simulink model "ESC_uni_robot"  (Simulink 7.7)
settings: Solver=ode3  StartTime=starttime  StopTime=stoptime  FixedStep=stepsize  RelTol=1e-3
PreLoadFcn:
  | load('ESC_GUI_params_uni')
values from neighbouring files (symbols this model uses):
  Kd = 60    [sim_run_multi.m]    (also in sim_run_uni.m)
  Kp = 3000    [sim_run_multi.m]    (also in sim_run_uni.m)
  noise_max = value    [ESC_GUI_multi.m]    (also in ESC_GUI_uni.m; sim_run_multi.m = 0.01; sim_run_uni.m = 0.2)
  obj_mean = -0.4    [sim_run_uni.m]
  obj_var = 0.27    [sim_run_uni.m]
  switch_noise = 1    [ESC_GUI_multi.m]    (also in ESC_GUI_uni.m; sim_run_multi.m; sim_run_uni.m)
  switch_optimizer = method_no+1    [ESC_GUI_multi.m]    (also in ESC_GUI_uni.m = method_no; sim_run_multi.m = 4; sim_run_uni.m = 1)
  x0 = [0;0]    [sim_run_multi.m]    (also in sim_run_uni.m = 0)
undefined symbols (not defined in the file or in its folder): approx, nn, perturb, sm_periodic
libraries: roblocks x8, simulink x1, commnoisgen2 x1

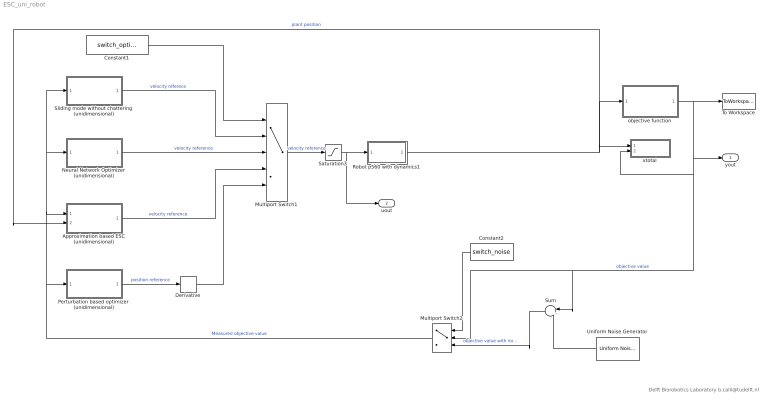
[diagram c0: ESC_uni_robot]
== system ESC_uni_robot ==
  note: Delft Biorobotics Laboratory b.calli@tudelft.nl
  Approximation based ESC (unidimensional) : Subsystem  mask{K_grad=approx.K_grad, sampling=approx.sampling, data_size=approx.data_size, poly_degree=approx.poly_degree, vel_init=approx.vel_init, lpf_constant=approx.filter_constant}
      mask prompts: data_size "Data size"; poly_degree "Poly degree"; vel_init "Initial velocity"; lpf_constant "Filter Constant"
  Constant1 : Constant  Value=switch_optimizer
  Constant2 : Constant  Value=switch_noise
  Derivative : Derivative
  Multiport Switch1 : MultiPortSwitch  Inputs=4  zeroidx=off
  Multiport Switch2 : MultiPortSwitch  Inputs=2  zeroidx=off
  Neural Network Optimizer (unidimensional) : Subsystem  mask{M=nn.M, A=nn.A, B=nn.B, ddelta=nn.ddelta, delta=nn.delta, mpd_init=nn.mpd_init}
      mask prompts: mpd_init "Minimum peak detector initial value"
  Perturbation based optimizer (unidimensional) : Subsystem  mask{high_pass_pole=perturb.high_pass_pole, sine_amp=perturb.sine_amp, sine_freq=perturb.sine_freq, low_pass_pole=perturb.low_pass_pole, corr_gain=perturb.corr_gain, comp_zero=perturb.comp_zero, comp_pole=perturb.comp_pole}
      mask prompts: high_pass_pole "High Pass Filter Pole"; sine_amp "Perturbation Signal Amplitude"; sine_freq "Perturbation Signal Frequency"; low_pass_pole "Low Pass Filter Pole"; corr_gain "Correction Gain"; comp_zero "Compensator Zero"; comp_pole "Compensator Pole"
  Robot p560 with dynamics1 : Subsystem
  Saturation3 : Saturate  UpperLimit=1  LowerLimit=-1
  Sliding mode without chattering (unidimensional) : Subsystem  mask{alpha=sm_periodic.alpha, rho=sm_periodic.rho, k=sm_periodic.k, g_init=sm_periodic.g_init}
      mask prompts: g_init "initial g"
  Sum : Sum  Inputs=|++
  To Workspace : ToWorkspace  VariableName=y  SampleTime=-1  SaveFormat=Structure With Time
  Uniform Noise Generator : commnoisgen2/Uniform Noise Generator  SystemSampleTime=-1  low=-noise_max  up=noise_max  seed=31  Ts=0.001  frameBased=off  sampPerFrame=1  orient=off  outDataType=double
  objective function : Stateflow chart  TreatAsAtomicUnit=on
  xtotal : Subsystem
  yout : Outport
  uout : Outport  Port=2
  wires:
  Robot p560 with dynamics1/1(x) -> objective function/1(x), Approximation based ESC (unidimensional)/2(x), xtotal/1(x)  "plant position"
  Multiport Switch1/1 -> Saturation3/1  "velocity reference"
  Neural Network Optimizer (unidimensional)/1(xdot_ref) -> Multiport Switch1/3  "velocity reference"
  Sliding mode without chattering (unidimensional)/1(xdot_ref) -> Multiport Switch1/2  "velocity referece"
  Constant1/1 -> Multiport Switch1/1
  Approximation based ESC (unidimensional)/1(xdot_ref) -> Multiport Switch1/4  "velocity reference"
  objective function/1(y) -> To Workspace/1, Multiport Switch2/2, Sum/1, xtotal/2(y), yout/1  "objective value"
  Uniform Noise Generator/1 -> Sum/2
  Sum/1 -> Multiport Switch2/3  "objective value with noise"
  Constant2/1 -> Multiport Switch2/1
  Perturbation based optimizer (unidimensional)/1(xref) -> Derivative/1  "position reference"
  Derivative/1 -> Multiport Switch1/5
  Multiport Switch2/1 -> Sliding mode without chattering (unidimensional)/1(y), Neural Network Optimizer (unidimensional)/1(y), Approximation based ESC (unidimensional)/1(y), Perturbation based optimizer (unidimensional)/1(y)  "Measured objective value"
  Saturation3/1 -> Robot p560 with dynamics1/1(xref), uout/1

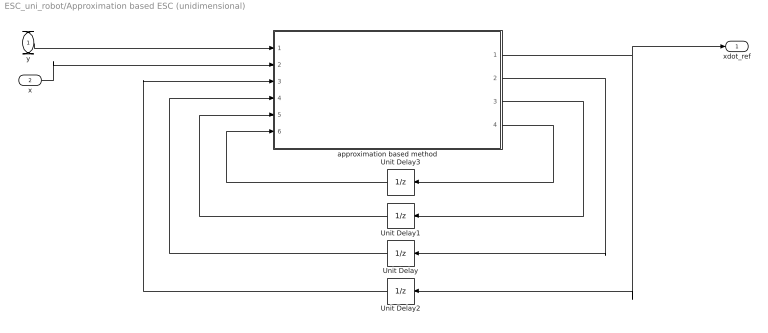
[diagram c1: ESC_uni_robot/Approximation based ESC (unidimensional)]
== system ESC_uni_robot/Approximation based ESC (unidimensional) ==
  y : Inport
  x : Inport  Port=2
  Unit Delay : UnitDelay  X0=zeros(1,data_size)  SampleTime=-1
  Unit Delay1 : UnitDelay  X0=zeros(1,data_size)  SampleTime=-1
  Unit Delay2 : UnitDelay  SampleTime=-1
  Unit Delay3 : UnitDelay  SampleTime=-1
  approximation based method : Stateflow chart  TreatAsAtomicUnit=on
  xdot_ref : Outport
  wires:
  approximation based method/2(x_data_arr_out) -> Unit Delay/1
  Unit Delay/1 -> approximation based method/4(x_data_arr)
  approximation based method/3(y_data_arr_out) -> Unit Delay1/1
  Unit Delay1/1 -> approximation based method/5(y_data_arr)
  y/1 -> approximation based method/1(y_data_in)
  x/1 -> approximation based method/2(x_data_in)
  approximation based method/1(xdot_ref) -> Unit Delay2/1, xdot_ref/1
  approximation based method/4(sample_out) -> Unit Delay3/1
  Unit Delay2/1 -> approximation based method/3(xdot_ref_in)
  Unit Delay3/1 -> approximation based method/6(sample)

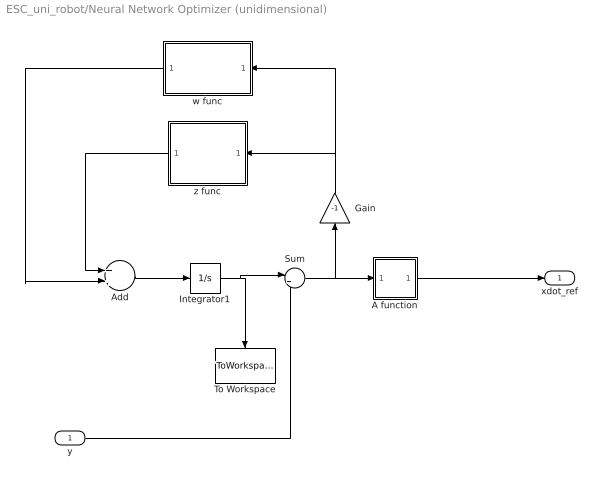
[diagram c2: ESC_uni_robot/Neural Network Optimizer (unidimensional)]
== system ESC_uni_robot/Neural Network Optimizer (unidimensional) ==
  y : Inport
  A function : Subsystem
  Add : Sum
  Gain : Gain  Gain=-1
  Integrator1 : Integrator  InitialCondition=mpd_init
  Sum : Sum  Inputs=|+-
  To Workspace : ToWorkspace  VariableName=yd_out  SampleTime=-1  SaveFormat=Structure With Time
  w func : Subsystem
  z func : Subsystem
  xdot_ref : Outport
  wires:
  Sum/1 -> Gain/1, A function/1(e)
  Gain/1 -> w func/1(e_minus), z func/1(e_minus)
  w func/1(w) -> Add/2
  z func/1(z) -> Add/1
  Add/1 -> Integrator1/1
  Integrator1/1 -> Sum/1, To Workspace/1
  A function/1(xdot) -> xdot_ref/1
  y/1 -> Sum/2

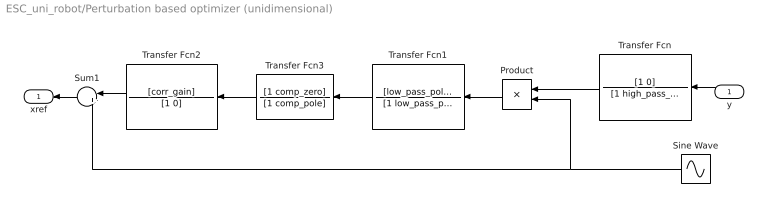
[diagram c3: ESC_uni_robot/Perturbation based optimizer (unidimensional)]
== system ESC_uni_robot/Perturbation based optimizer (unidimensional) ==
  y : Inport
  Product : Product
  Sine Wave : Sin  Amplitude=sine_amp  Frequency=sine_freq  SampleTime=0
  Sum1 : Sum  Inputs=|++
  Transfer Fcn : TransferFcn  Numerator=[1 0]  Denominator=[1 high_pass_pole]
  Transfer Fcn1 : TransferFcn  Numerator=[low_pass_pole]  Denominator=[1 low_pass_pole]
  Transfer Fcn2 : TransferFcn  Numerator=[corr_gain]  Denominator=[1 0]
  Transfer Fcn3 : TransferFcn  Numerator=[1 comp_zero]  Denominator=[1 comp_pole]
  xref : Outport
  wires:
  Transfer Fcn/1 -> Product/1
  Sine Wave/1 -> Product/2, Sum1/2
  Product/1 -> Transfer Fcn1/1
  Transfer Fcn1/1 -> Transfer Fcn3/1
  Transfer Fcn2/1 -> Sum1/1
  y/1 -> Transfer Fcn/1
  Sum1/1 -> xref/1
  Transfer Fcn3/1 -> Transfer Fcn2/1

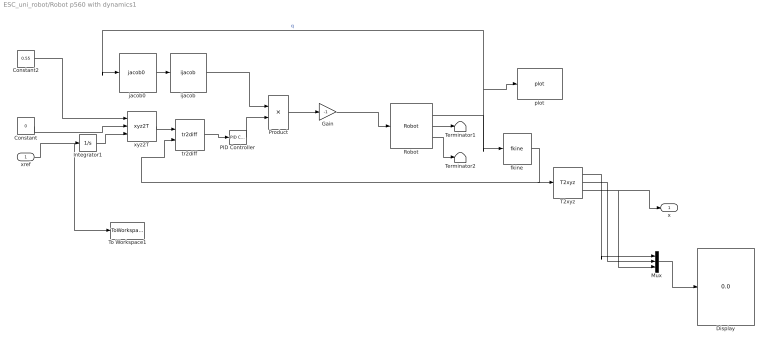
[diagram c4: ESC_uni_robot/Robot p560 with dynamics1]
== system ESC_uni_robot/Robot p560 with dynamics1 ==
  xref : Inport
  Constant : Constant  Value=0
  Constant2 : Constant  Value=0.55
  Display : Display
  Gain : Gain  Gain=-1
  Integrator1 : Integrator  InitialCondition=x0
  Mux : Mux  Inputs=3
  PID Controller : simulink/Continuous/PID Controller  SystemSampleTime=-1  Controller=PID  TimeDomain=Continuous-time  SampleTime=1  IntegratorMethod=Forward Euler  FilterMethod=Forward Euler  Form=Parallel  P=[Kp Kp Kp Kp Kp Kp]  I=[0 0 0 0 0 0]  D=[Kd Kd Kd Kd Kd Kd]  N=100  InitialConditionSource=internal  InitialConditionForIntegrator=0  InitialConditionForFilter=0  ExternalReset=none  LimitOutput=off  UpperSaturationLimit=inf  LowerSaturationLimit=-inf  LinearizeAsGain=off  AntiWindupMode=none  Kb=1  TrackingMode=off  Kt=1  PParamMin=[]  PParamMax=[]  IParamMin=[]  IParamMax=[]  DParamMin=[]  DParamMax=[]  NParamMin=[]  NParamMax=[]  KbParamMin=[]  KbParamMax=[]  KtParamMin=[]  KtParamMax=[]  POutMin=[]  POutMax=[]  IOutMin=[]  IOutMax=[]  DOutMin=[]  DOutMax=[]  NOutMin=[]  NOutMax=[]  KbOutMin=[]  KbOutMax=[]  KtOutMin=[]  KtOutMax=[]  IntegratorOutMin=[]  IntegratorOutMax=[]  FilterOutMin=[]  FilterOutMax=[]  SumOutMin=[]  SumOutMax=[]  SumI1OutMin=[]  SumI1OutMax=[]  SumI2OutMin=[]  SumI2OutMax=[]  SumI3OutMin=[]  SumI3OutMax=[]  SumDOutMin=[]  SumDOutMax=[]  SaturationOutMin=[]  SaturationOutMax=[]  IntegratorContinuousStateAttributes=''  IntegratorStateMustResolveToSignalObject=off  IntegratorRTWStateStorageClass=Auto  FilterContinuousStateAttributes=''  FilterStateMustResolveToSignalObject=off  FilterRTWStateStorageClass=Auto
  Product : Product  Multiplication=Matrix(*)
  Robot : roblocks/Robot  SystemSampleTime=-1  robot=p560  q0="[0.2763    0.9125    2.9359         0    2.4348   -0.2763]"
  T2xyz : roblocks/T2xyz  SystemSampleTime=-1
  Terminator1 : Terminator
  Terminator2 : Terminator
  To Workspace1 : ToWorkspace  VariableName=u_out  SampleTime=-1  SaveFormat=Structure With Time
  fkine : roblocks/fkine  SystemSampleTime=-1  robot=p560
  ijacob : roblocks/ijacob  SystemSampleTime=-1
  jacob0 : roblocks/jacob0   SystemSampleTime=-1  robot=p560
  plot : roblocks/plot  SystemSampleTime=-1  robot=p560
  tr2diff : roblocks/tr2diff  SystemSampleTime=-1  robot=robot
  xyz2T : roblocks/xyz2T  SystemSampleTime=-1
  x : Outport
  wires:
  Robot/1 -> fkine/1, jacob0/1, plot/1  "q"
  tr2diff/1 -> PID Controller/1
  xyz2T/1 -> tr2diff/1
  fkine/1 -> T2xyz/1, tr2diff/2
  jacob0/1 -> ijacob/1
  ijacob/1 -> Product/1
  Product/1 -> Gain/1
  Gain/1 -> Robot/1
  PID Controller/1 -> Product/2
  Robot/2 -> Terminator1/1
  Robot/3 -> Terminator2/1
  xref/1 -> Integrator1/1, To Workspace1/1
  T2xyz/1 -> Mux/1
  T2xyz/2 -> Mux/2
  T2xyz/3 -> Mux/3, x/1
  Mux/1 -> Display/1
  Constant/1 -> xyz2T/2
  Constant2/1 -> xyz2T/1
  Integrator1/1 -> xyz2T/3

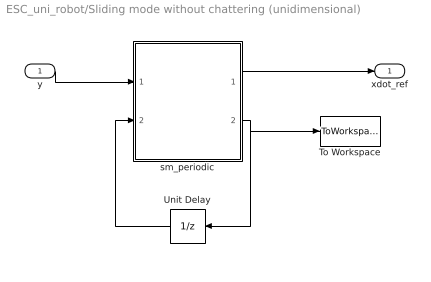
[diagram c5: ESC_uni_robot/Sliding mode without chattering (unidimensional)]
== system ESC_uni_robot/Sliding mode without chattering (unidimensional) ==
  y : Inport
  To Workspace : ToWorkspace  VariableName=g_sm_out  SampleTime=-1  SaveFormat=Structure With Time
  Unit Delay : UnitDelay  X0=g_init  SampleTime=-1
  sm_periodic : Stateflow chart  TreatAsAtomicUnit=on
  xdot_ref : Outport
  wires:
  y/1 -> sm_periodic/1(y)
  sm_periodic/1(u) -> xdot_ref/1
  sm_periodic/2(g_out) -> Unit Delay/1, To Workspace/1
  Unit Delay/1 -> sm_periodic/2(g_in)

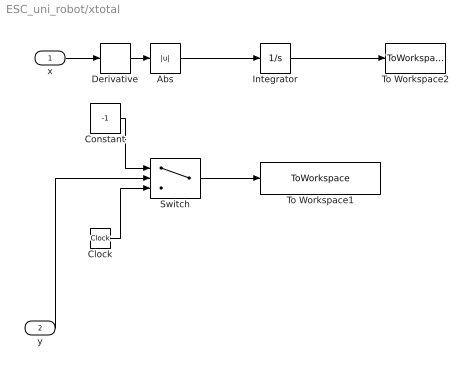
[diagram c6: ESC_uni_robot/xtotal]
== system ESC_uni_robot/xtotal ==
  x : Inport
  y : Inport  Port=2
  Abs : Abs
  Clock : Clock
  Constant : Constant  Value=-1
  Derivative : Derivative
  Integrator : Integrator
  Switch : Switch  Threshold=1.05
  To Workspace1 : ToWorkspace  VariableName=peak_time_detector  SampleTime=-1  SaveFormat=Array
  To Workspace2 : ToWorkspace  VariableName=x_total  SampleTime=-1  SaveFormat=Array
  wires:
  y/1 -> Switch/2
  Clock/1 -> Switch/3
  Switch/1 -> To Workspace1/1
  Constant/1 -> Switch/1
  x/1 -> Derivative/1
  Integrator/1 -> To Workspace2/1
  Abs/1 -> Integrator/1
  Derivative/1 -> Abs/1

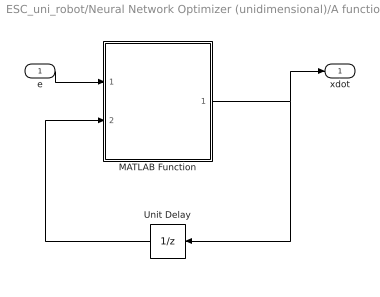
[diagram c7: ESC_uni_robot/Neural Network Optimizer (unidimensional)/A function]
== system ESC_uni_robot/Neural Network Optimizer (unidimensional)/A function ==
  e : Inport
  MATLAB Function : Stateflow chart  TreatAsAtomicUnit=on
  Unit Delay : UnitDelay  X0=-A  SampleTime=-1
  xdot : Outport
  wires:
  Unit Delay/1 -> MATLAB Function/2(x_dot_pre)
  MATLAB Function/1(xdot) -> xdot/1, Unit Delay/1
  e/1 -> MATLAB Function/1(e)

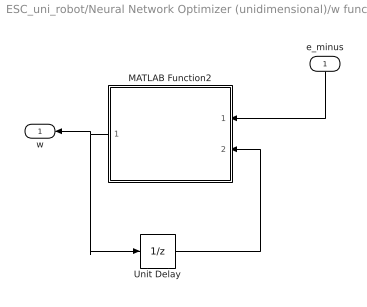
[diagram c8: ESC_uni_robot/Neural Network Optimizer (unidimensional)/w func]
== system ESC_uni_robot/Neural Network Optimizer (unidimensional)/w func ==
  e_minus : Inport
  MATLAB Function2 : Stateflow chart  TreatAsAtomicUnit=on
  Unit Delay : UnitDelay  SampleTime=-1
  w : Outport
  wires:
  e_minus/1 -> MATLAB Function2/1(e_minus)
  Unit Delay/1 -> MATLAB Function2/2(w_pre)
  MATLAB Function2/1(w) -> w/1, Unit Delay/1

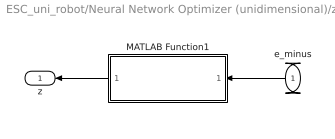
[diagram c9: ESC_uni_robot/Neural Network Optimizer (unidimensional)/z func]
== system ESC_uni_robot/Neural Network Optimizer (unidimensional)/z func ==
  e_minus : Inport
  MATLAB Function1 : Stateflow chart  TreatAsAtomicUnit=on
  z : Outport
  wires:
  e_minus/1 -> MATLAB Function1/1(e_minus)
  MATLAB Function1/1(z) -> z/1

== matlab function Neural Network Optimizer
(unidimensional)/A function/MATLAB Function ==
function xdot = nn_ESC(e,x_dot_pre,A,ddelta)
%#codegen

if( e<-ddelta )
    xdot = -A;
elseif(e>ddelta)
    xdot = A;
else
    xdot = x_dot_pre;
end

end

== matlab function Approximation based ESC
(unidimensional)/approximation based method ==
function [xdot_ref,x_data_arr_out,y_data_arr_out, sample_out] = approx_based_method(y_data_in, x_data_in, xdot_ref_in, x_data_arr, y_data_arr,K_grad, sample, sampling, poly_degree, data_size, vel_init, lpf_constant)
%#codegen
if(mod(sample,sampling) == 0)
    sample_out = sample+1;
    x_data_arr = circshift(x_data_arr,1);
    y_data_arr = circshift(y_data_arr,1);
    x_data_arr(1) = x_data_in;
    y_data_arr(1) = y_data_in;
    
    V = zeros(data_size,poly_degree+1);

    % forming the vandermonde matrix 
    for i=1:data_size
        for j=1:poly_degree+1
            V(i,j) = x_data_arr(i)^(poly_degree-j+1);
        end
    end
   
    c = pinv(V)*y_data_arr;     % calculating coefficients
    x = x_data_arr(1);
    
    % calculating gradient
    grad_val = 0; 
    for i = 1:poly_degree
        grad_val = grad_val+c(i)*(poly_degree+1-i)*x.^(poly_degree-i);
    end
    
    
    if (sample<sampling*data_size)      % collecting first set for approximation with a constant velocity
        xdot_ref = vel_init;
    else                                % calculating velocity references otherwise
        xdot_ref = -K_grad*grad_val;
        if (xdot_ref~=xdot_ref)         % if the result of the approximation is NAN because of an ill-poised data set, keep the previous the velocity reference.
            xdot_ref = xdot_ref_in;
        end
    end
    
    % apply lowpass filtering for output
    if(xdot_ref~=vel_init)
        xdot_ref = lpf_constant * xdot_ref + ( 1.0 - lpf_constant ) * xdot_ref_in;
    end
    
    x_data_arr_out = x_data_arr;
    y_data_arr_out = y_data_arr;
else
    sample_out = sample+1;
    x_data_arr_out = x_data_arr;
    y_data_arr_out = y_data_arr;
    xdot_ref = xdot_ref_in;
end

== matlab function Neural Network Optimizer
(unidimensional)/z func/MATLAB Function1 ==
function z = zfunc(e_minus,M)
%#codegen
if(e_minus>0)
    z = 0;
else
    z = -M;
end
end

== matlab function Neural Network Optimizer
(unidimensional)/w func/MATLAB Function2 ==
function w = wfunc(e_minus,w_pre,B,delta)
%#codegen
if(e_minus<-delta)
    w = 0;
elseif (e_minus>delta)
    w = B;
else
    w = w_pre;
end
end

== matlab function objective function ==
function y = objective_function(x, obj_mean, obj_var)
%#codegen

y=obj_func_uni(x,obj_mean,obj_var);

== matlab function Sliding mode without chattering
(unidimensional)/sm_periodic ==
function [u,g_out]  = sm_periodic(y,g_in,alpha, k, rho)
%#codegen

g_out = g_in-rho;
s = y-g_out;

u = k*sign(sin(pi/alpha*s));
